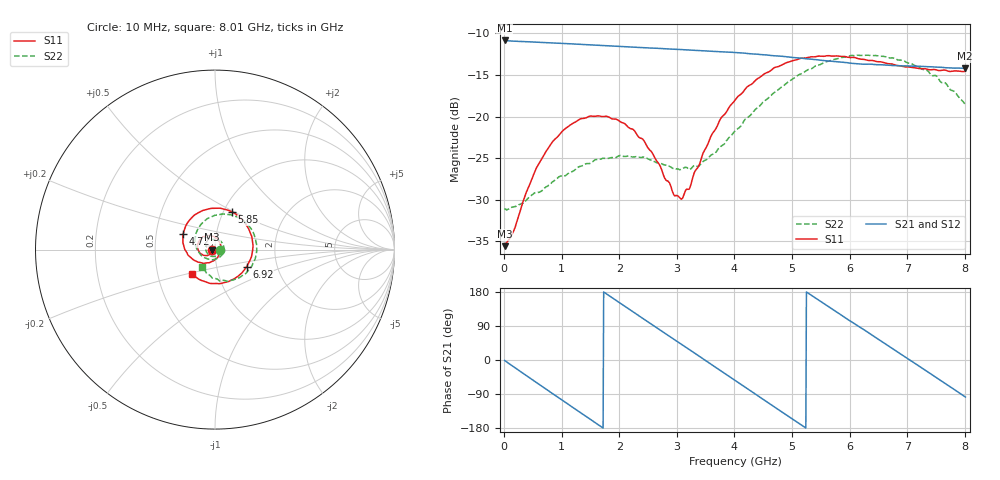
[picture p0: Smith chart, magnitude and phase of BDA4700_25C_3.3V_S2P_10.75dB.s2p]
!Agilent Technologies,E5071B,MY42404982,A.09.10
!Date: Mon Oct 20 18:07:31 2025
!Data & Calibration Information:
!Freq	S11:SOLT2(ON)	S21:SOLT2(ON)	S12:SOLT2(ON)	S22:SOLT2(ON)
# Hz S RI R 50
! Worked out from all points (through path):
!   801 points, 10 MHz to 8.01 GHz, reference 50 ohm
!   highest |S21| = -10.86 dB at 10 MHz (marker M1); lowest = -14.2 dB at 8 GHz (marker M2)
!   group delay of S21, straight-line fit = 283 ps
!   lowest |S11| = -35.6 dB at 10 MHz (marker M3), VSWR 1.03, Z = 48.4 - j0.115 ohm
!   |S11| at or under -10 dB: start of sweep to end of sweep
!   |S22| runs from -31.2 to -12.6 dB; largest |S21 - S12| = 0.0033
!   S11 on the Smith chart (normalised r, x): 10 MHz: 0.97, -0.00; 4.72 GHz: 0.69, +0.12; 5.85 GHz: 1.10, +0.48; 6.92 GHz: 1.40, -0.28; 8.01 GHz: 0.75, -0.21
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1e7  -0.0166 -0.00119  0.2864 -0.00645  0.2864 -0.00651  0.028 -0.0014
1.6e8  -0.0176 -0.0101  0.2712 -0.084  0.2711 -0.084  0.0271 -0.00897
3.3e8  -0.023 -0.0204  0.2309 -0.1622  0.2307 -0.1624  0.0228 -0.0196
7.2e8  -0.0507 -0.0336  0.0678 -0.2697  0.068 -0.2697  -0.000986 -0.0375
1.35e9  -0.0969 0.00749  -0.2116 -0.1699  -0.2116 -0.17  -0.0499 -0.00719
1.93e9  -0.0664 0.07  -0.2471 0.0953  -0.2471 0.0954  -0.0267 0.0497
2.32e9  -0.0169 0.0745  -0.126 0.2278  -0.1259 0.2279  0.0171 0.0546
2.68e9  0.0229 0.0471  0.0352 0.2544  0.0348 0.2542  0.0467 0.0239
2.95e9  0.0325 0.00925  0.1471 0.2069  0.1467 0.2064  0.0479 -0.00764
3.09e9  0.0299 -0.0116  0.193 0.1628  0.1915 0.1638  0.0417 -0.0245
3.54e9  -0.0174 -0.0662  0.2466 -0.0239  0.2467 -0.0243  -0.00689 -0.0556
4.01e9  -0.1081 -0.0633  0.1437 -0.1955  0.144 -0.195  -0.074 -0.0345
4.36e9  -0.1639 -0.00564  0.00221 -0.2373  0.00211 -0.2379  -0.1081 0.0204
4.72e9  -0.1789 0.085  -0.1377 -0.186  -0.1369 -0.1869  -0.1035 0.0965
5.35e9  -0.0611 0.2199  -0.2169 0.0407  -0.2171 0.0395  0.0201 0.1937
5.85e9  0.0959 0.2086  -0.1034 0.1855  -0.1029 0.1853  0.1612 0.158
6.28e9  0.1908 0.108  0.0467 0.2009  0.0494 0.1995  0.2292 0.0444
6.68e9  0.2064 -0.0233  0.1633 0.121  0.1637 0.1208  0.2134 -0.0732
6.92e9  0.1762 -0.0947  0.1966 0.0445  0.1964 0.0435  0.174 -0.131
7.46e9  0.0324 -0.1891  0.1478 -0.1325  0.1479 -0.1327  0.0323 -0.1733
8e9  -0.1236 -0.14  -0.023 -0.1933  -0.0226 -0.1935  -0.0698 -0.0965
8.01e9  -0.126 -0.1383  -0.0265 -0.1929  -0.0258 -0.193  -0.0709 -0.0944
